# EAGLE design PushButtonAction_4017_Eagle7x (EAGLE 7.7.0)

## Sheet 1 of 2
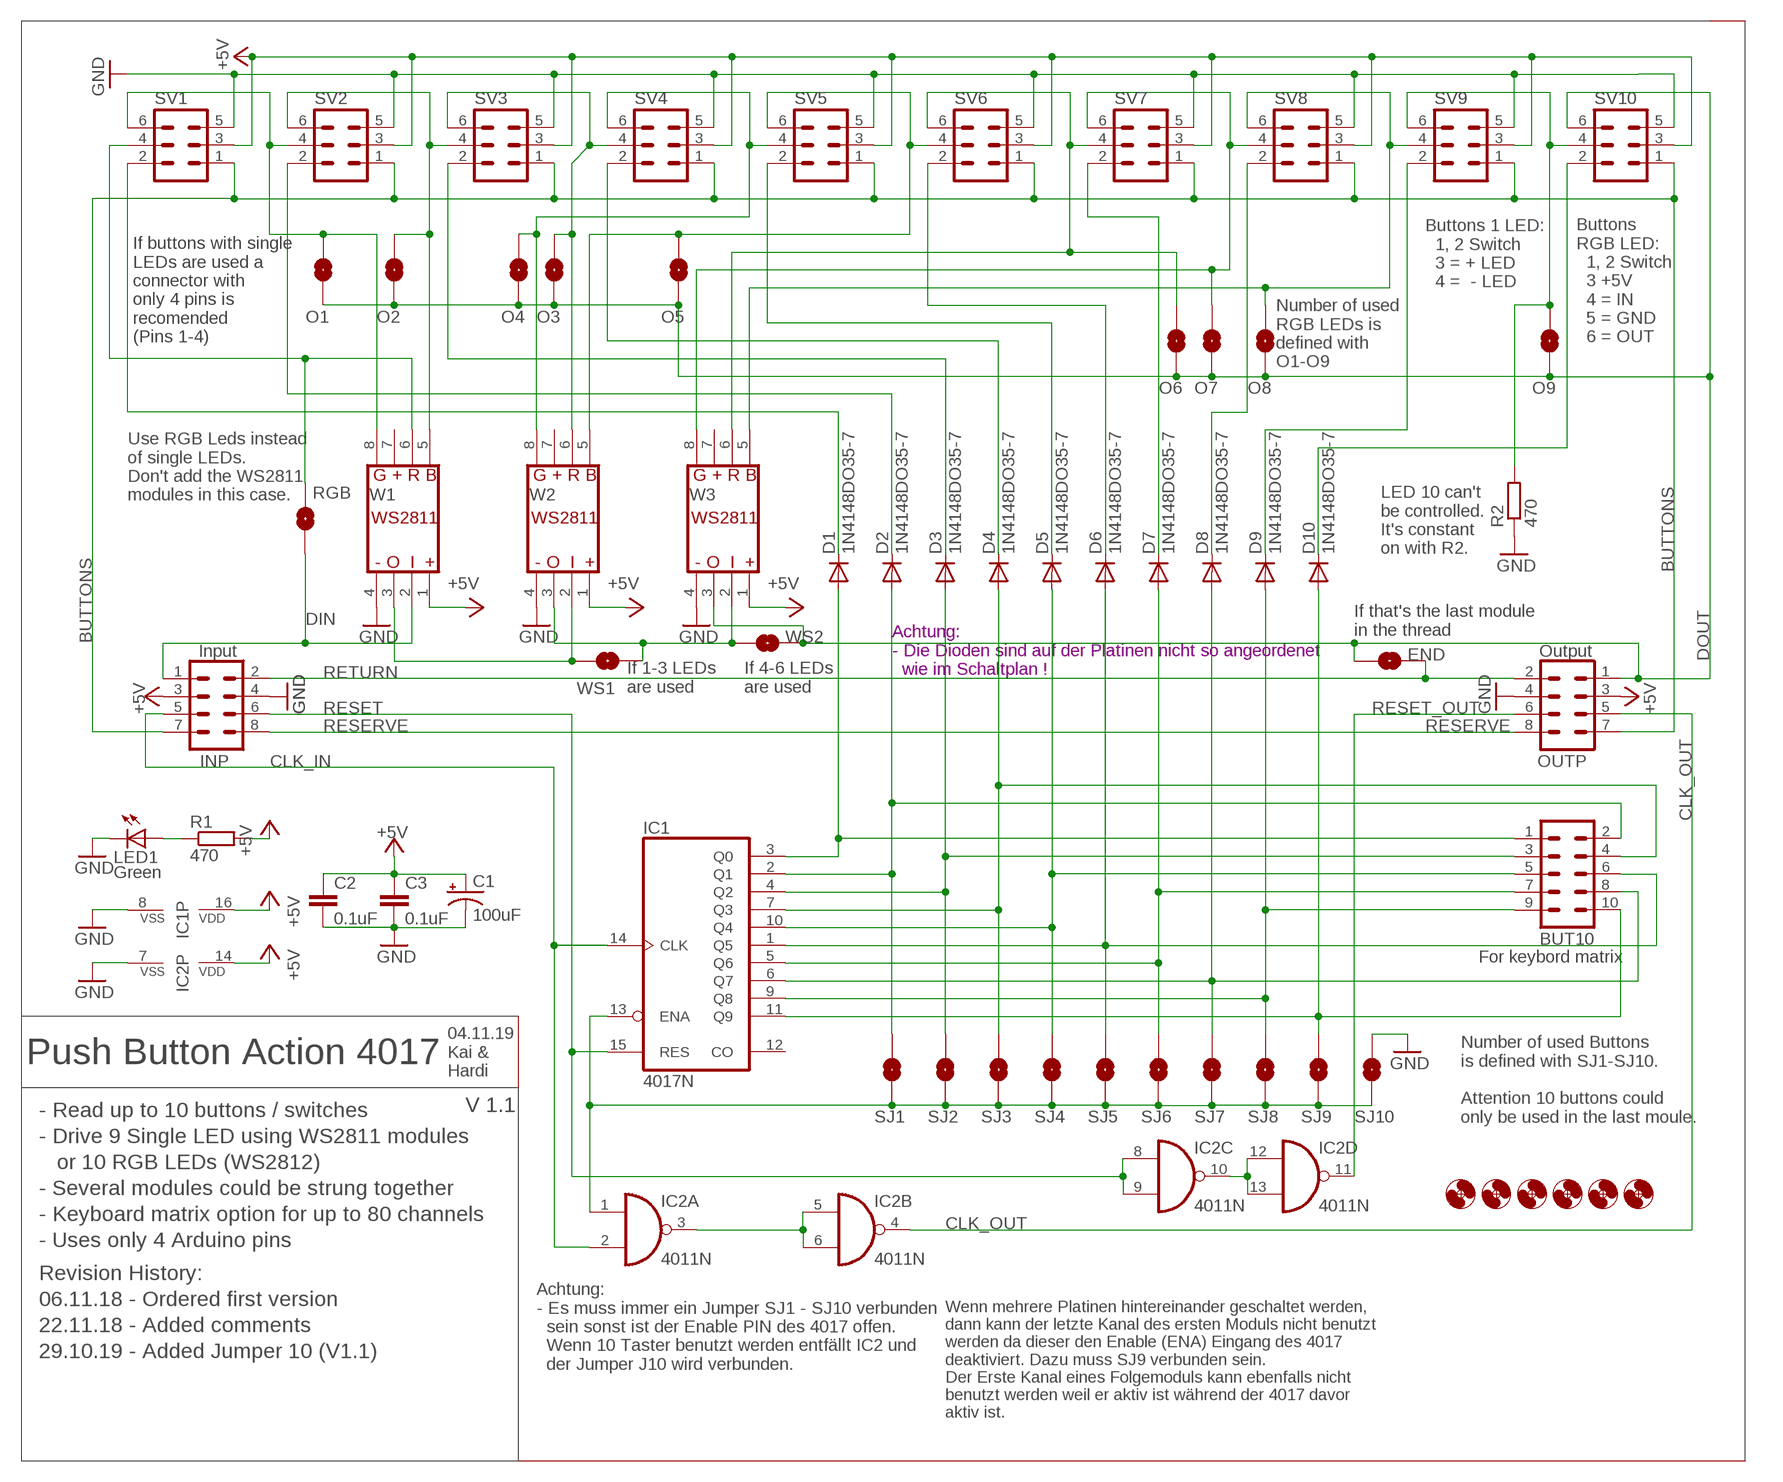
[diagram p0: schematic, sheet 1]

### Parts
BUT10  CON-HARTING-ML_ML10  [CON-HARTING-ML_ML10]
C1  100uF  100UF-25V-20%(PTH)  [CPOL-RADIAL-100UF-25V]
C2  0.1uF  0.1UF-50V-20%(PTH)KIT-EZ  [CAP-PTH-SMALL-KIT]
C3  0.1uF  0.1UF-50V-20%(PTH)KIT-EZ  [CAP-PTH-SMALL-KIT]
D1  1N4148DO35-7  [DO35-7]
D2  1N4148DO35-7  [DO35-7]
D3  1N4148DO35-7  [DO35-7]
D4  1N4148DO35-7  [DO35-7]
D5  1N4148DO35-7  [DO35-7]
D6  1N4148DO35-7  [DO35-7]
D7  1N4148DO35-7  [DO35-7]
D8  1N4148DO35-7  [DO35-7]
D9  1N4148DO35-7  [DO35-7]
D10  1N4148DO35-7  [DO35-7]
END  SOLDERJUMPERNO  [SJ_2S-NO]
H1  MOUNT-HOLE3.0  [3,0]
H2  MOUNT-HOLE3.0  [3,0]
H3  MOUNT-HOLE3.0  [3,0]
H4  MOUNT-HOLE3.0  [3,0]
H5  MOUNT-HOLE3.0  [3,0]
H6  MOUNT-HOLE3.0  [3,0]
IC1  4017N  [DIL16]
IC2  4011N  [DIL14]
INP  CON-HARTING-ML_ML08  [CON-HARTING-ML_ML08]
LED1  Green  LED3MM  [LED3MM]
O1  SOLDERJUMPERNO  [SJ_2S-NO]
O2  SOLDERJUMPERNO  [SJ_2S-NO]
O3  SOLDERJUMPERNO  [SJ_2S-NO]
O4  SOLDERJUMPERNO  [SJ_2S-NO]
O5  SOLDERJUMPERNO  [SJ_2S-NO]
O6  SOLDERJUMPERNO  [SJ_2S-NO]
O7  SOLDERJUMPERNO  [SJ_2S-NO]
O8  SOLDERJUMPERNO  [SJ_2S-NO]
O9  SOLDERJUMPERNO  [SJ_2S-NO]
OUTP  CON-HARTING-ML_ML08  [CON-HARTING-ML_ML08]
R1  470  R-EU_0207/2V  [0207/2V]
R2  470  R-EU_0204/5  [0204/5]
RGB  SOLDERJUMPERNO  [SJ_2S-NO]
SJ1  SOLDERJUMPERNO  [SJ_2S-NO]
SJ2  SOLDERJUMPERNO  [SJ_2S-NO]
SJ3  SOLDERJUMPERNO  [SJ_2S-NO]
SJ4  SOLDERJUMPERNO  [SJ_2S-NO]
SJ5  SOLDERJUMPERNO  [SJ_2S-NO]
SJ6  SOLDERJUMPERNO  [SJ_2S-NO]
SJ7  SOLDERJUMPERNO  [SJ_2S-NO]
SJ8  SOLDERJUMPERNO  [SJ_2S-NO]
SJ9  SOLDERJUMPERNO  [SJ_2S-NO]
SJ10  SOLDERJUMPERNO  [SJ_2S-NO]
SV1  CON-HARTING-ML_ML6  [CON-HARTING-ML_ML6]
SV2  CON-HARTING-ML_ML6  [CON-HARTING-ML_ML6]
SV3  CON-HARTING-ML_ML6  [CON-HARTING-ML_ML6]
SV4  CON-HARTING-ML_ML6  [CON-HARTING-ML_ML6]
SV5  CON-HARTING-ML_ML6  [CON-HARTING-ML_ML6]
SV6  CON-HARTING-ML_ML6  [CON-HARTING-ML_ML6]
SV7  CON-HARTING-ML_ML6  [CON-HARTING-ML_ML6]
SV8  CON-HARTING-ML_ML6  [CON-HARTING-ML_ML6]
SV9  CON-HARTING-ML_ML6  [CON-HARTING-ML_ML6]
SV10  CON-HARTING-ML_ML6  [CON-HARTING-ML_ML6]
W1  WS28115V  [WS2811_WS2811_5V]
W2  WS28115V  [WS2811_WS2811_5V]
W3  WS28115V  [WS2811_WS2811_5V]
WS1  SOLDERJUMPERNO  [SJ_2S-NO]
WS2  SOLDERJUMPERNO  [SJ_2S-NO]

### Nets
+5V: C1.1(+) C2.1 C3.1 IC1.16(VDD) IC2.14(P:VDD) INP.3 OUTP.3 R1.2 SV1.3 SV2.3 SV3.3 SV4.3 SV5.3 SV6.3 SV7.3 SV8.3 SV9.3 SV10.3 W1.1 W2.1 W3.1
BUTTONS: INP.7 OUTP.7 SV1.1 SV2.1 SV3.1 SV4.1 SV5.1 SV6.1 SV7.1 SV8.1 SV9.1 SV10.1
CLK_IN: IC1.14(CLK) IC2.2(A:I1) INP.5
CLK_OUT: IC2.4(B:O) OUTP.5
DIN: INP.1 RGB.1 W1.2
DOUT: END.2 O1.1 O2.1 O3.1 O4.1 O5.1 O6.1 O7.1 O8.1 O9.1 OUTP.1 SV10.6 W3.3 WS2.1
GND: C1.2(-) C2.2 C3.2 IC1.8(VSS) IC2.7(P:VSS) INP.4 LED1.K(C) OUTP.4 R2.1 SJ10.2 SV1.5 SV2.5 SV3.5 SV4.5 SV5.5 SV6.5 SV7.5 SV8.5 SV9.5 SV10.5 W1.4 W2.4 W3.4
N$1: IC2.3(A:O) IC2.5(B:I0) IC2.6(B:I1)
N$2: IC1.13(ENA) IC2.1(A:I0) SJ1.1 SJ2.1 SJ3.1 SJ4.1 SJ5.1 SJ6.1 SJ7.1 SJ8.1 SJ9.1 SJ10.1
N$3: IC2.10(C:O) IC2.12(D:I0) IC2.13(D:I1)
N$4: RGB.2 SV1.4 W1.6
N$5: BUT10.10 D10.A IC1.11(Q9) SJ9.2
N$6: D1.C SV1.2
N$7: W1.3 W2.2 WS1.1
N$8: O5.2 SV5.6 SV6.4 W2.5
N$9: D2.C SV2.2
N$10: D3.C SV3.2
N$11: BUT10.2 D2.A IC1.2(Q1) SJ1.2
N$12: BUT10.3 D3.A IC1.4(Q2) SJ2.2
N$13: BUT10.4 D4.A IC1.7(Q3) SJ3.2
N$14: BUT10.5 D5.A IC1.10(Q4) SJ4.2
N$15: BUT10.6 D6.A IC1.1(Q5) SJ5.2
N$16: BUT10.7 D7.A IC1.5(Q6) SJ6.2
N$17: BUT10.8 D8.A IC1.6(Q7) SJ7.2
N$18: BUT10.9 D9.A IC1.9(Q8) SJ8.2
N$19: D4.C SV4.2
N$20: D5.C SV5.2
N$21: LED1.A R1.1
N$22: W2.3 W3.2 WS1.2 WS2.2
N$23: D6.C SV6.2
N$25: D8.C SV8.2
N$26: D9.C SV9.2
N$27: D10.C SV10.2
N$35: BUT10.1 D1.A IC1.3(Q0)
N$45: O1.2 SV1.6 SV2.4 W1.8
N$46: O2.2 SV2.6 SV3.4 W1.5
N$49: O4.2 SV4.6 SV5.4 W2.8
N$51: O3.2 SV3.6 SV4.4 W2.6
N$54: O6.2 SV6.6 SV7.4 W3.6
N$56: O7.2 SV7.6 SV8.4 W3.8
N$57: O8.2 SV8.6 SV9.4 W3.5
N$58: O9.2 R2.2 SV9.6 SV10.4
O6: D7.C SV7.2
RESERVE: INP.8 OUTP.8
RESET: IC1.15(RES) IC2.8(C:I0) IC2.9(C:I1) INP.6
RESET_OUT: IC2.11(D:O) OUTP.6
RETURN: END.1 INP.2 OUTP.2
Unconnected: IC1.12(CO) W1.7 W2.7 W3.7

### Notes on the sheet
- Buttons 1 LED:
    1, 2 Switch
    3 = + LED
    4 =  - LED
- If buttons with single 
  LEDs are used a 
  connector with
  only 4 pins is 
  recomended
  (Pins 1-4)
- Buttons
  RGB LED:
    1, 2 Switch
    3 +5V
    4 = IN
    5 = GND
    6 = OUT
- Number of used
  RGB LEDs is 
  defined with 
  O1-O9
- Use RGB Leds instead
  of single LEDs.
  Don't add the WS2811
  modules in this case.
- LED 10 can't
  be controlled.
  It's constant
  on with R2.
- Achtung:
  - Die Dioden sind auf der Platinen nicht so angeordenet
    wie im Schaltplan !
- If that's the last module 
  in the thread
- Input | Output
- If 1-3 LEDs
  are used
- If 4-6 LEDs
  are used
- For keybord matrix
- Push Button Action 4017
- 04.11.19
  Kai & 
  Hardi
- V 1.1
- Number of used Buttons
  is defined with SJ1-SJ10.
  
  Attention 10 buttons could
  only be used in the last moule.
- - Read up to 10 buttons / switches
  - Drive 9 Single LED using WS2811 modules
     or 10 RGB LEDs (WS2812)
  - Several modules could be strung together
  - Keyboard matrix option for up to 80 channels
  - Uses only 4 Arduino pins
- Revision History:
  06.11.18 - Ordered first version
  22.11.18 - Added comments
  29.10.19 - Added Jumper 10 (V1.1)
- Achtung:
  - Es muss immer ein Jumper SJ1 - SJ10 verbunden
    sein sonst ist der Enable PIN des 4017 offen.
    Wenn 10 Taster benutzt werden entfällt IC2 und 
    der Jumper J10 wird verbunden.
- Wenn mehrere Platinen hintereinander geschaltet werden,
  dann kann der letzte Kanal des ersten Moduls nicht benutzt
  werden da dieser den Enable (ENA) Eingang des 4017
  deaktiviert. Dazu muss SJ9 verbunden sein.
  Der Erste Kanal eines Folgemoduls kann ebenfalls nicht
  benutzt werden weil er aktiv ist während der 4017 davor
  aktiv ist.

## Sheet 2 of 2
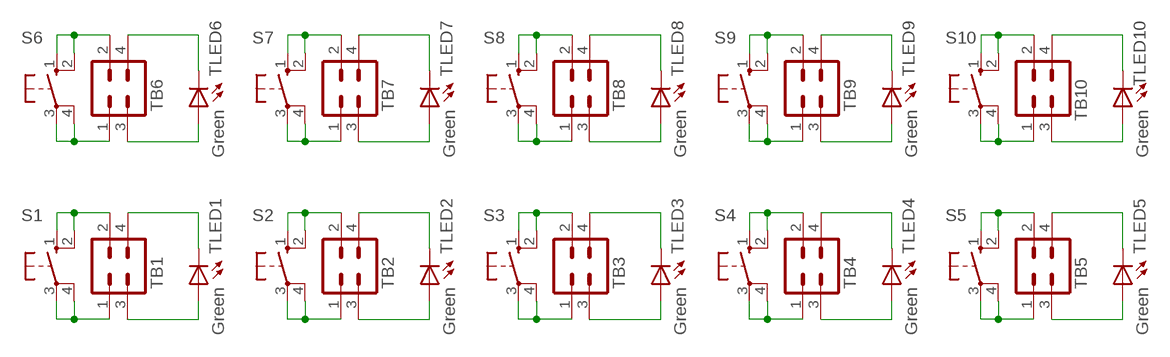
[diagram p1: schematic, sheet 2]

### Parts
S1  10-XX  [B3F-10XX]
S2  10-XX  [B3F-10XX]
S3  10-XX  [B3F-10XX]
S4  10-XX  [B3F-10XX]
S5  10-XX  [B3F-10XX]
S6  10-XX  [B3F-10XX]
S7  10-XX  [B3F-10XX]
S8  10-XX  [B3F-10XX]
S9  10-XX  [B3F-10XX]
S10  10-XX  [B3F-10XX]
TB1  CON-HARTING-ML_ML4ML4_FEMALE  [ML_ML4_FEMALE]
TB2  CON-HARTING-ML_ML4ML4_FEMALE  [ML_ML4_FEMALE]
TB3  CON-HARTING-ML_ML4ML4_FEMALE  [ML_ML4_FEMALE]
TB4  CON-HARTING-ML_ML4ML4_FEMALE  [ML_ML4_FEMALE]
TB5  CON-HARTING-ML_ML4ML4_FEMALE  [ML_ML4_FEMALE]
TB6  CON-HARTING-ML_ML4ML4_FEMALE  [ML_ML4_FEMALE]
TB7  CON-HARTING-ML_ML4ML4_FEMALE  [ML_ML4_FEMALE]
TB8  CON-HARTING-ML_ML4ML4_FEMALE  [ML_ML4_FEMALE]
TB9  CON-HARTING-ML_ML4ML4_FEMALE  [ML_ML4_FEMALE]
TB10  CON-HARTING-ML_ML4ML4_FEMALE  [ML_ML4_FEMALE]
TLED1  Green  LED_LED3MM  [LED_LED3MM]
TLED2  Green  LED_LED3MM  [LED_LED3MM]
TLED3  Green  LED_LED3MM  [LED_LED3MM]
TLED4  Green  LED_LED3MM  [LED_LED3MM]
TLED5  Green  LED_LED3MM  [LED_LED3MM]
TLED6  Green  LED_LED3MM  [LED_LED3MM]
TLED7  Green  LED_LED3MM  [LED_LED3MM]
TLED8  Green  LED_LED3MM  [LED_LED3MM]
TLED9  Green  LED_LED3MM  [LED_LED3MM]
TLED10  Green  LED_LED3MM  [LED_LED3MM]

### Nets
N$24: S1.1(S) S1.2(S1) TB1.2
N$28: S1.3(P) S1.4(P1) TB1.1
N$29: TB1.3 TLED1.A
N$30: TB1.4 TLED1.K(C)
N$31: S2.1(S) S2.2(S1) TB2.2
N$32: S2.3(P) S2.4(P1) TB2.1
N$33: TB2.3 TLED2.A
N$34: TB2.4 TLED2.K(C)
N$36: S3.1(S) S3.2(S1) TB3.2
N$37: S3.3(P) S3.4(P1) TB3.1
N$38: TB3.3 TLED3.A
N$39: TB3.4 TLED3.K(C)
N$40: S4.1(S) S4.2(S1) TB4.2
N$41: S4.3(P) S4.4(P1) TB4.1
N$42: TB4.3 TLED4.A
N$43: TB4.4 TLED4.K(C)
N$44: S5.1(S) S5.2(S1) TB5.2
N$47: S5.3(P) S5.4(P1) TB5.1
N$48: TB5.3 TLED5.A
N$50: TB5.4 TLED5.K(C)
N$52: S6.1(S) S6.2(S1) TB6.2
N$53: S6.3(P) S6.4(P1) TB6.1
N$55: TB6.3 TLED6.A
N$59: TB6.4 TLED6.K(C)
N$60: S7.1(S) S7.2(S1) TB7.2
N$61: S7.3(P) S7.4(P1) TB7.1
N$62: TB7.3 TLED7.A
N$63: TB7.4 TLED7.K(C)
N$64: S8.1(S) S8.2(S1) TB8.2
N$65: S8.3(P) S8.4(P1) TB8.1
N$66: TB8.3 TLED8.A
N$67: TB8.4 TLED8.K(C)
N$68: S9.1(S) S9.2(S1) TB9.2
N$69: S9.3(P) S9.4(P1) TB9.1
N$70: TB9.3 TLED9.A
N$71: TB9.4 TLED9.K(C)
N$72: S10.1(S) S10.2(S1) TB10.2
N$73: S10.3(P) S10.4(P1) TB10.1
N$74: TB10.3 TLED10.A
N$75: TB10.4 TLED10.K(C)

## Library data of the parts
BUT10 = PushButtonAction_4017_2:CON-HARTING-ML_ML10: HARTING; OC_FARNELL: unknown; OC_NEWARK: unknown
C1 = SparkFun-Capacitors:100UF-25V-20%(PTH): CAP-08439; PROD_ID: CAP-08439
C2 C3 = SparkFun-Capacitors:0.1UF-50V-20%(PTH): CAP-08370; PROD_ID: CAP-08370
D1-D10 = diode:1N4148: DIODE
END O1-O9 RGB SJ1-SJ10 WS1 WS2 = SparkFun-Retired:SOLDERJUMPER: Solder Jumper
H1-H6 = holes:MOUNT-HOLE: MOUNTING HOLE with drill center marker
IC1 = 40xx:4017: COUNTER/DIVIDER
IC2 = 40xx:4011: Quad 2-input NAND; SPICEPREFIX: J
INP OUTP = PushButtonAction_4017_2:CON-HARTING-ML_ML08: Modified by Hardi; OC_FARNELL: unknown; OC_NEWARK: unknown
LED1 = led:LED: LED
R1 R2 = rcl:R-EU_: RESISTOR, European symbol; SPICEPREFIX: R
S1-S10 = switch-omron:10-XX: OMRON SWITCH; MPN: B3F-1000; OC_FARNELL: 176432; OC_NEWARK: 36M3542
SV1-SV10 = PushButtonAction_4017_4:CON-HARTING-ML_ML6: HARTING; OC_FARNELL: unknown; OC_NEWARK: unknown
TB1-TB10 = RGB-LED-Verteiler:CON-HARTING-ML_ML4
TLED1-TLED10 = Sound_MP3-TF-16P_and_WS2811:LED_LED: LED
W1-W3 = PushButtonAction_4017_2:WS2811: Modified by Hardi

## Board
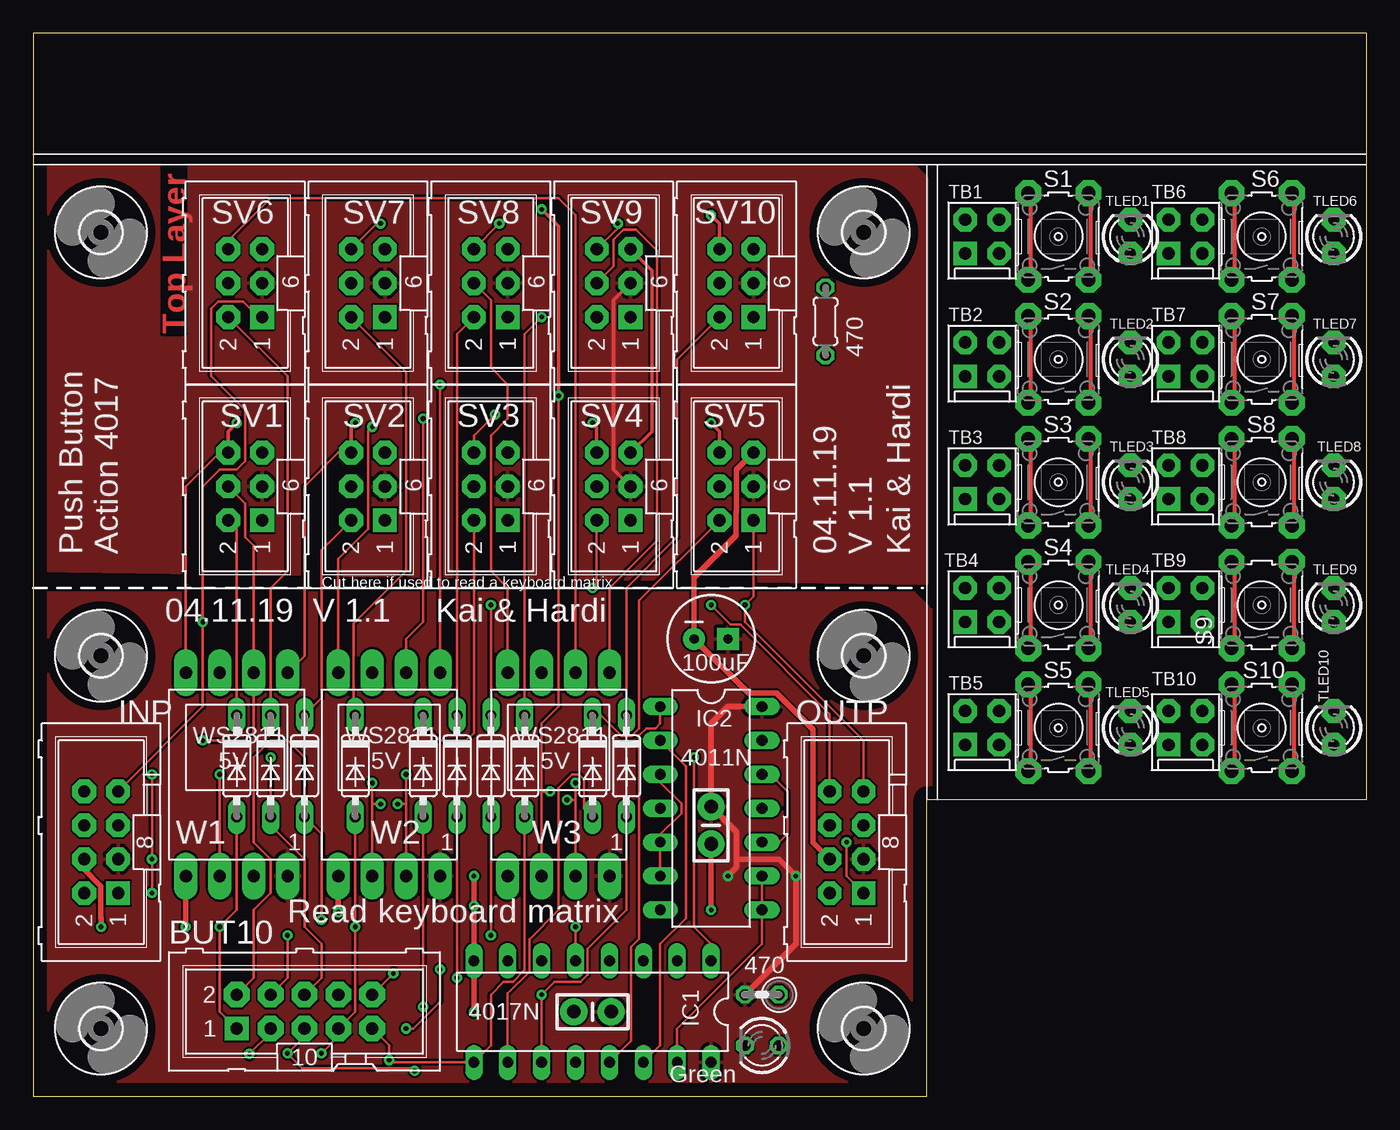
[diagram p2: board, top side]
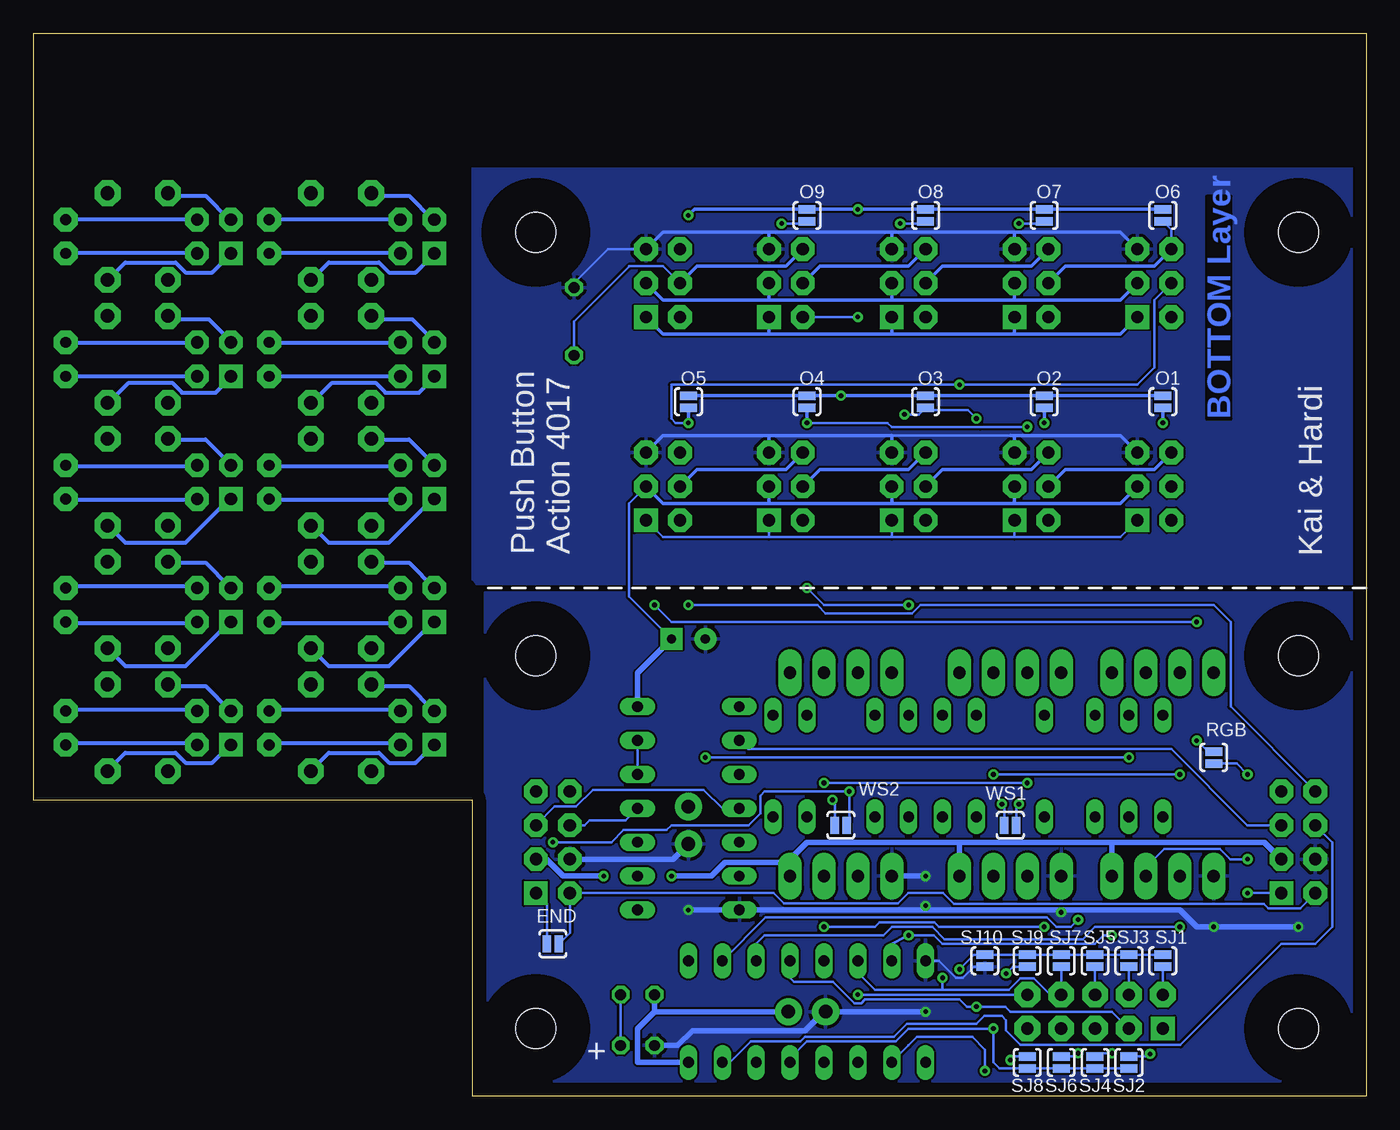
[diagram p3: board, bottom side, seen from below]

Size 99.9 x 79.68 mm. Coordinates in mm from the lower left corner, seen from the top.
Outline: 0,0 66.98,0 66.98,22.23 99.9,22.23 99.9,79.68 0,79.68 0,0
Copper layers (1*16): Top 0.035mm / dielectric 1.5mm / Bottom 0.035mm
Design rules "default *": minimum track width 6mil, minimum drill 0.35mm, track to track 6mil, track to pad 6mil, pad to pad 6mil, via to via 6mil, smd to smd 6mil, copper to edge 40mil, drill to drill 6mil, minimum pad ring 10mil, minimum via ring 8mil, stop-mask expansion 4mil, vias tented up to drill 0mil, thermal gap 10mil

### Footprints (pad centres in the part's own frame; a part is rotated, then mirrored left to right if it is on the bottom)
CON-HARTING-ML_ML10 = drill 0.914 pad 1.778 square: 1 -5.08,-1.27 | drill 0.914 pad 1.93 octagon: 2 -5.08,1.27; 3 -2.54,-1.27; 4 -2.54,1.27; 5 0,-1.27; 6 0,1.27; 7 2.54,-1.27; 8 2.54,1.27; 9 5.08,-1.27; 10 5.08,1.27
CPOL-RADIAL-100UF-25V = drill 0.7 pad 1.651 square: 1 1.27,0 | drill 0.7 pad 1.651: 2 -1.27,0
CAP-PTH-SMALL-KIT = drill 1.016 pad 2.032: 1 -1.397,0; 2 1.397,0
DO35-7 = drill 0.813 long: A 3.81,0; C -3.81,0
SJ_2S-NO = smd 0.635 x 1.27: 1 -0.45,0; 2 0.45,0
3,0 = hole 3: 0,0
DIL16 = drill 0.813 long: 1 -8.89,-3.81; 2 -6.35,-3.81; 3 -3.81,-3.81; 4 -1.27,-3.81; 5 1.27,-3.81; 6 3.81,-3.81; 7 6.35,-3.81; 8 8.89,-3.81; 9 8.89,3.81; 10 6.35,3.81; 11 3.81,3.81; 12 1.27,3.81; 13 -1.27,3.81; 14 -3.81,3.81; 15 -6.35,3.81; 16 -8.89,3.81
DIL14 = drill 0.813 long: 1 -7.62,-3.81; 2 -5.08,-3.81; 3 -2.54,-3.81; 4 0,-3.81; 5 2.54,-3.81; 6 5.08,-3.81; 7 7.62,-3.81; 8 7.62,3.81; 9 5.08,3.81; 10 2.54,3.81; 11 0,3.81; 12 -2.54,3.81; 13 -5.08,3.81; 14 -7.62,3.81
CON-HARTING-ML_ML08 = drill 0.914 pad 1.778 square: 1 -5.08,-1.27 | drill 0.914 pad 1.778 octagon: 2 -5.08,1.27; 3 -2.54,-1.27; 4 -2.54,1.27; 5 0,-1.27; 6 0,1.27; 7 2.54,-1.27; 8 2.54,1.27
LED3MM = drill 0.813 octagon: A -1.27,0; K 1.27,0
0207/2V = drill 0.813 octagon: 1 -1.27,0; 2 1.27,0
0204/5 = drill 0.813 octagon: 1 -2.54,0; 2 2.54,0
B3F-10XX = drill 1.016 pad 1.93 octagon: 1 -3.251,2.261; 2 3.251,2.261; 3 -3.251,-2.261; 4 3.251,-2.261
CON-HARTING-ML_ML6 = drill 0.914 pad 1.778 square: 1 -2.54,-1.27 | drill 0.914 pad 1.778 octagon: 2 -2.54,1.27; 3 0,-1.27; 4 0,1.27; 5 2.54,-1.27; 6 2.54,1.27
ML_ML4_FEMALE = drill 0.914 pad 1.778 square: 1 -2.54,-1.27 | drill 0.914 pad 1.778 octagon: 2 -2.54,1.27; 3 0,-1.27; 4 0,1.27
LED_LED3MM = drill 0.813 pad 1.778 octagon: A -1.27,0; K 1.27,0
WS2811_WS2811_5V = drill 0.914 pad 1.778 long: 1 2.54,-5.08; 2 0,-5.08; 3 -2.54,-5.08; 4 -5.08,-5.08; 5 2.54,10.16; 6 0,10.16; 7 -2.54,10.16; 8 -5.08,10.16

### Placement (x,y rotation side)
BUT10  20.32,6.35 0 top
C1  50.8,34.29 0 top
C2  50.8,20.32 270 top
C3  41.91,6.35 180 top
D1  15.24,24.77 270 top
D2  20.32,24.77 270 top
D3  29.21,24.77 270 top
D4  34.29,24.77 270 top
D5  41.91,24.77 270 top
D6  17.78,24.77 270 top
D7  24.13,24.77 270 top
D8  31.75,24.77 270 top
D9  36.83,24.77 270 top
D10  44.45,24.77 270 top
END  60.96,11.43 180 bottom
H1  62.23,5.08 90 top
H2  5.08,5.08 90 top
H3  5.08,64.77 90 top
H4  62.23,64.77 90 top
H5  5.08,33.02 90 top
H6  62.23,33.02 90 top
IC1  41.91,6.35 180 top
IC2  50.8,21.59 270 top
INP  5.08,20.32 90 top
LED1  54.61,3.81 180 top
O1  15.24,52.07 270 bottom
O2  24.13,52.07 270 bottom
O3  33.02,52.07 270 bottom
O4  41.91,52.07 270 bottom
O5  50.8,52.07 270 bottom
O6  15.24,66.04 270 bottom
O7  24.13,66.04 270 bottom
O8  33.02,66.04 270 bottom
O9  41.91,66.04 270 bottom
OUTP  60.96,20.32 90 top
R1  54.61,7.62 180 top
R2  59.37,58.09 270 top
RGB  11.43,25.4 90 bottom
S1  76.83,64.45 90 top
S2  76.83,55.24 90 top
S3  76.83,46.04 90 top
S4  76.83,36.83 90 top
S5  76.83,27.62 90 top
S6  92.08,64.45 90 top
S7  92.08,55.24 90 top
S8  92.08,46.04 90 top
S9  92.08,36.83 90 top
S10  92.08,27.62 90 top
SJ1  15.24,10.16 270 bottom
SJ2  17.78,2.54 90 bottom
SJ3  17.78,10.16 270 bottom
SJ4  20.32,2.54 90 bottom
SJ5  20.32,10.16 270 bottom
SJ6  22.86,2.54 90 bottom
SJ7  22.86,10.16 270 bottom
SJ8  25.4,2.54 90 bottom
SJ9  25.4,10.16 270 bottom
SJ10  28.57,10.16 270 bottom
SV1  15.88,45.72 90 top
SV2  25.08,45.72 90 top
SV3  34.29,45.72 90 top
SV4  43.5,45.72 90 top
SV5  52.7,45.72 90 top
SV6  15.88,60.96 90 top
SV7  25.08,60.96 90 top
SV8  34.29,60.96 90 top
SV9  43.5,60.96 90 top
SV10  52.7,60.96 90 top
TB1  72.39,64.45 0 top
TB2  72.39,55.24 0 top
TB3  72.39,46.04 0 top
TB4  72.39,36.83 0 top
TB5  72.39,27.62 0 top
TB6  87.63,64.45 0 top
TB7  87.63,55.24 0 top
TB8  87.63,46.04 0 top
TB9  87.63,36.83 0 top
TB10  87.63,27.62 0 top
TLED1  82.23,64.45 90 top
TLED2  82.23,55.24 90 top
TLED3  82.23,46.04 90 top
TLED4  82.23,36.83 90 top
TLED5  82.23,27.62 90 top
TLED6  97.47,64.45 90 top
TLED7  97.47,55.24 90 top
TLED8  97.47,46.04 90 top
TLED9  97.47,36.83 90 top
TLED10  97.47,27.62 90 top
W1  16.51,21.59 0 top
W2  27.94,21.59 0 top
W3  40.64,21.59 0 top
WS1  26.67,20.32 0 bottom
WS2  39.37,20.32 180 bottom

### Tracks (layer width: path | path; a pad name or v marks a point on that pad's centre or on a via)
+5V  (via drill 0.35)
  Top 0.254: SV9.3 43.5,59.69 43.5,46.99 SV4.3
  Top 0.406: IC2.14 52.07,29.21 50.8,27.94 C2.1 52.7,19.81 52.7,17.78 | R1.2 57.15,11.43 v57.15,16.51 55.88,17.78 52.7,17.78 | 52.7,17.78 52.7,17.14 v52.07,16.51
  Bottom 0.203: SV5.3 55.24,44.45 55.24,37.47 C1.1
  Bottom 0.254: SV6.3 18.41,59.69 26.35,59.69 | 26.35,59.69 35.56,59.69 | 35.56,59.69 44.77,59.69 | 44.77,59.69 52.7,59.69 SV10.3 | SV7.3 26.35,59.69 | SV8.3 35.56,59.69 | SV9.3 44.77,59.69 | SV1.3 18.41,44.45 26.35,44.45 | 26.35,44.45 35.56,44.45 | 35.56,44.45 44.77,44.45 | 44.77,44.45 52.7,44.45 SV5.3 | SV2.3 26.35,44.45 | SV3.3 35.56,44.45 | SV4.3 44.77,44.45
  Bottom 0.406: 19.05,19.05 7.62,19.05 INP.3 | 19.05,19.05 30.48,19.05 | 30.48,19.05 41.91,19.05 43.18,17.78 | OUTP.3 61.45,17.78 60.21,16.54 57.17,16.54 v57.15,16.51 | v52.07,16.51 49.09,16.51 48.07,17.53 43.43,17.53 43.18,17.78 | 53.34,6.35 R1.2 | C3.1 53.34,6.35 | 53.34,6.35 54.61,5.08 54.61,2.54 IC1.16 | C1.1 54.61,31.75 IC2.14 | W1.1 19.05,19.05 | W3.1 43.18,17.78 | W2.1 30.48,19.05
  pour Top: 0,0 67.31,0 67.31,36.51 66.04,37.78 0.95,37.78 0,1.27
  pour Top: 66.99,38.42 66.99,68.9 66.04,69.85 1.27,69.85 0,68.58 0,39.37
BUTTONS  (via drill 0.35)
  Top 0.203: INP.7 12.7,29.21 v12.7,35.56 12.7,45.72 13.97,46.99 15.24,46.99 15.88,47.62 15.88,51.44 13.34,53.98 13.34,59.05 13.84,59.56 15.71,59.56 16.86,58.42 SV6.1 | SV5.1 53.98,37.47 v53.34,36.83 53.34,35.56 62.23,26.67 OUTP.7
  Bottom 0.203: SV1.1 18.41,41.91 26.35,41.91 | 26.35,41.91 35.56,41.91 | 35.56,41.91 44.77,41.91 | 44.77,41.91 52.7,41.91 SV5.1 | SV2.1 26.35,41.91 | SV3.1 35.56,41.91 | SV4.1 44.77,41.91 | v12.7,35.56 52.07,35.56 v53.34,36.83
  Bottom 0.254: SV6.1 18.41,57.15 26.35,57.15 | 26.35,57.15 35.56,57.15 | 35.56,57.15 44.77,57.15 | 44.77,57.15 52.7,57.15 SV10.1 | SV7.1 26.35,57.15 | SV8.1 35.56,57.15 | SV9.1 44.77,57.15
CLK_IN
  Top 0.203: IC2.2 48.9,24.77 48.92,24.74 48.92,13.36 46.99,11.43 46.99,3.81 IC1.14
  Bottom 0.203: INP.5 8.89,20.32 14.6,26.03 46.35,26.03 IC2.2
CLK_OUT
  Bottom 0.203: IC2.4 48.26,21.59 49.66,22.99 57.95,22.99 59.22,21.72 60.83,21.72 OUTP.5
DIN  (via drill 0.35)
  Top 0.203: v8.89,15.24 v8.89,17.78 v8.89,24.13
  Bottom 0.203: INP.1 7.62,15.24 v8.89,15.24 | v8.89,17.78 10.2,17.78 10.96,18.54 15.11,18.54 16.51,17.14 W1.2 | v8.89,24.13 9.71,24.95 RGB.1
DOUT  (via drill 0.35)
  Top 0.203: OUTP.1 60.96,16.51 v60.96,19.05 | 38.1,22.86 38.1,27.94 39.37,29.21 v39.37,52.52 | 38.1,22.86 v38.74,22.86 | W3.3 38.1,22.86
  Top 0.254: SV10.6 51.44,65.41 v50.8,66.04 | v39.37,52.52 39.37,65.22 v38.1,66.49
  Bottom 0.203: OUTP.1 61.41,14.42 END.2 | WS2.1 38.74,20.5 v38.74,22.86 45.09,22.86 45.41,22.53 45.41,21.21 46.31,20.32 52.07,20.32 52.43,19.96 55.65,19.96 56.56,19.05 v60.96,19.05
  Bottom 0.254: O6.1 O7.1 O8.1 v38.1,66.49 O9.1 50.35,66.49 v50.8,66.04 | O1.1 O2.1 | O1.1 O3.1 | v39.37,52.52 35.56,52.52 O1.1 | v39.37,52.52 O4.1 | v39.37,52.52 O5.1
GND  (via drill 0.35)
  Top 0.254: SV9.5 46.35,61.91 46.35,49.85 SV4.5
  Top 0.406: v33.02,6.35 IC1.8 v33.02,14.29 v33.02,16.51 | INP.4 3.81,17 5.05,15.76 5.05,13.36 5.08,13.34 v5.08,12.7 | 22.86,13.65 v22.86,13.79 W2.4 | C2.2 v50.8,13.97 | SV5.5 52.7,46.99 52.7,43.81 52.68,43.79 52.68,42.03 49.53,38.88 C1.2 53.59,30.23 55.69,30.23 58.42,27.5 58.42,19.05 OUTP.4 | W1.4 v11.43,12.7
  Bottom 0.203: 35.56,49.53 26.67,49.53 | SV10.5 56.83,63.5 59.37,60.96 R2.1 | SJ10.2 29.4,9.71 30.22,8.89 30.74,8.89 32.01,10.16 IC1.8
  Bottom 0.254: SV6.5 18.41,64.77 26.35,64.77 | SV10.5 52.7,64.77 44.77,64.77 | 26.35,64.77 35.56,64.77 | 35.56,64.77 44.77,64.77 | 26.35,64.77 SV7.5 | 35.56,64.77 SV8.5 | 44.77,64.77 SV9.5 | SV1.5 18.41,49.53 26.35,49.53 | 26.35,49.53 26.67,49.53 | 44.77,49.53 35.56,49.53 SV3.5 | 44.77,49.53 52.7,49.53 SV5.5 | SV2.5 26.35,49.53 | SV4.5 44.77,49.53
  Bottom 0.406: 33.02,13.97 IC2.7 v50.8,13.97 | v33.02,14.29 33.02,13.97 | 33.02,13.97 22.86,13.97 | 22.86,13.97 13.97,13.97 12.7,12.7 v11.43,12.7 v5.08,12.7 | v22.86,13.79 22.86,13.97 | v33.02,6.35 C3.2 40.64,6.35 42.06,4.93 50.51,4.93 51.63,3.81 LED1.K | OUTP.4 51.94,17.78 C2.2 | W3.4 v33.02,16.51
  pour Bottom: 0,0 66.04,0 66.04,37.78 0,37.78
  pour Bottom: 0,38.42 66.67,38.42 66.99,38.73 66.99,69.53 0.95,69.53
N$1
  Top 0.203: IC2.6 IC2.5 46.99,19.64 48.56,21.21 48.56,21.97 46.99,23.54 IC2.3
N$2  (via drill 0.35)
  Top 0.203: IC1.13 44.81,4.17 44.81,11.2 45.41,11.81 45.41,27.05 45.95,27.58 46.63,27.58 46.99,27.94 IC2.1 | v30.48,9.53 30.48,7.09 28.47,5.08 v27.94,5.08
  Bottom 0.203: SJ1.1 SJ3.1 SJ5.1 SJ7.1 SJ9.1 SJ10.1 29.39,10.61 v30.48,9.53 | SJ2.1 SJ4.1 SJ6.1 SJ8.1 27.49,2.09 27.94,2.54 v27.94,5.08 34.29,5.08 35.26,4.12 41.91,4.12 43.18,2.85 IC1.13
N$3
  Top 0.203: IC2.10 55.88,19.05 56.52,19.68 56.52,22.86 55.24,24.13 IC2.12
  Bottom 0.203: IC2.12 IC2.13
N$4  (via drill 0.35)
  Top 0.203: v12.7,26.67 15.88,26.67 16.51,27.3 W1.6 16.51,41.27 15.88,41.91 15.88,44.45 SV1.4
  Bottom 0.203: RGB.2 11.88,25.85 v12.7,26.67
N$5  (via drill 0.35)
  Top 0.203: IC1.11 v38.1,7.62 39.06,8.59 41.02,8.59 41.55,9.12 41.55,11.07 44.45,13.97 D10.A | BUT10.10 v26.99,9.21
  Bottom 0.203: BUT10.10 v38.1,7.62 | v26.99,9.21 26.48,9.71 SJ9.2
N$6
  Top 0.203: D1.C 15.24,42.55 SV1.2
N$7  (via drill 0.35)
  Top 0.203: 27.94,21.91 v27.94,24.13 | v27.3,21.91 27.94,21.91 | W1.3 v13.97,24.13 | W2.2 27.94,21.91
  Bottom 0.203: v13.97,24.13 v27.94,24.13 | WS1.1 27.12,21.72 v27.3,21.91
N$8  (via drill 0.35)
  Top 0.203: W2.5 v30.48,53.34
  Top 0.254: SV5.6 51.44,49.85 v50.8,50.48
  Bottom 0.203: v50.8,50.48 51.75,50.48 52.07,50.8 52.07,53.34 v30.48,53.34 17.14,53.34 15.88,54.61 15.88,59.69 SV6.4
  Bottom 0.254: v50.8,50.48 O5.2
N$9
  Top 0.203: D2.C 21.59,29.84 21.59,40.96 SV2.2
N$10
  Top 0.203: SV3.2 33.02,27.26 32.43,26.67 30.48,26.67 29.21,27.94 D3.C
N$11  (via drill 0.35)
  Top 0.203: BUT10.2 16.51,8.89 16.51,13.97 17.78,15.24 17.78,17.78 16.51,19.05 16.51,25.4 17.78,26.67 19.05,26.67 20.32,25.4 D2.A 21.59,19.68 v21.59,13.24
  Bottom 0.203: BUT10.2 SJ1.2 | IC1.2 45.01,13.41 23.95,13.41 23.24,12.7 22.13,12.7 v21.59,13.24
N$12  (via drill 0.35)
  Top 0.203: D3.A v29.21,6.72 | v16.19,3.17 17.78,4.76 BUT10.3
  Bottom 0.203: IC1.4 43.18,8.89 42.88,8.59 39.96,8.59 38.36,6.99 37.84,6.99 37.56,7.26 30.48,7.26 29.93,6.72 v29.21,6.72 27.04,6.72 26.67,6.35 19.05,6.35 BUT10.3 | SJ2.2 16.38,2.99 v16.19,3.17
N$13  (via drill 0.35)
  Top 0.203: BUT10.4 19.05,8.89 v19.05,12.06 | v34.29,12.06 D4.A
  Bottom 0.203: BUT10.4 SJ3.2 | v34.29,12.06 34.54,11.94 | 34.54,11.94 35.56,11.43 IC1.7 | v19.05,12.06 19.68,12.06 20.32,11.43 31.75,11.43 32.38,12.06 34.42,12.06 34.54,11.94
N$14  (via drill 0.35)
  Top 0.203: IC1.10 35.56,7.7 37.19,9.33 37.19,11.79 39.37,13.97 39.37,23.12 40.38,24.13 40.9,24.13 41.27,23.76 41.27,21.59 D5.A | BUT10.5 20.32,4.5 v19.05,3.23 19.05,3.17 20.14,2.09 26.67,2.09 28.39,2.09 v28.57,1.91
  Bottom 0.203: IC1.10 34.29,3.81 33.66,4.45 29.53,4.45 28.57,3.49 v28.57,1.91 | v19.05,3.23 20.08,3.23 SJ4.2
N$15  (via drill 0.35)
  Top 0.203: BUT10.6 21.59,8.89 21.59,11.43 20.32,12.7 20.32,17.78 17.78,20.32 D6.A v17.78,25.4 | IC1.1 50.8,11.43 49.53,12.7 v49.53,25.4
  Bottom 0.203: BUT10.6 SJ5.2 | v49.53,25.4 v17.78,25.4
N$16  (via drill 0.35)
  Top 0.203: D7.A v24.13,12.7 24.13,6.35 BUT10.7 22.86,4.5 v21.59,3.23 | v40.64,12.7 IC1.5
  Bottom 0.203: v24.13,12.7 32.01,12.7 32.37,13.06 36.47,13.06 36.83,12.7 v40.64,12.7 | SJ6.2 21.77,2.99 21.59,3.17 v21.59,3.23
N$17  (via drill 0.35)
  Top 0.203: v31.75,8.89 D8.A
  Bottom 0.203: SJ7.2 BUT10.8 23.68,7.62 24.89,8.84 25.91,8.84 26.77,7.98 31.75,7.98 | 31.75,7.98 36.83,7.98 38.1,9.25 IC1.6 | 31.75,7.98 v31.75,8.89
N$18  (via drill 0.35)
  Top 0.203: D9.A 36.83,9.48 35.94,8.59 35.26,8.59 34.29,7.62 34.29,3.81 IC1.9 26.67,2.54 v26.67,2.72 26.67,3.81 BUT10.9
  Bottom 0.203: v26.67,2.72 26.4,2.99 SJ8.2
N$19  (via drill 0.35)
  Top 0.203: D4.C v34.29,36.83 | SV4.2 42.23,38.42 v41.91,38.1
  Bottom 0.203: v34.29,36.83 40.64,36.83 v41.91,38.1
N$20
  Top 0.203: SV5.2 45.41,37.16 45.41,27.59 44.83,27 44.07,27 42.5,28.57 D5.C
N$21
  Bottom 0.203: LED1.A R1.1
N$22  (via drill 0.35)
  Top 0.203: v40.64,23.5 40.64,22.23 | 25.4,21.91 v25.4,23.5 | v40.01,22.23 40.64,22.23 | v26.04,21.91 25.4,21.91 | W2.3 25.4,21.91 | W3.2 40.64,22.23
  Bottom 0.203: v25.4,23.5 v40.64,23.5 | WS2.2 39.82,22.04 v40.01,22.23 | WS1.2 26.22,21.72 v26.04,21.91
N$23
  Top 0.203: D6.C 17.78,38.1 19.05,39.37 19.05,53.98 SV6.2
N$24
  Top 0.305: S1.1 74.75,61.25 74.75,67.5 S1.2
  Bottom 0.305: TB1.2 70,65.75 71.75,67.5 74.5,67.5 S1.2
N$25
  Top 0.203: D8.C 31.75,57.15 SV8.2
N$26  (via drill 0.35)
  Top 0.203: D9.C 36.83,57.15 v38.1,58.42
  Bottom 0.203: v38.1,58.42 SV9.2
N$27
  Top 0.203: D10.C 44.45,38.1 48.26,41.91 48.26,55.24 SV10.2
N$28
  Top 0.305: S1.4 79.25,67.5 79.25,61.25 S1.3
  Bottom 0.305: TB1.1 70,63 71.25,61.75 73.25,61.75 74,62.5 77.75,62.5 79,61.25 S1.3
N$29
  Bottom 0.305: TB1.3 72.5,63.25 82,63.25 TLED1.A
N$30
  Bottom 0.305: TB1.4 72.5,65.75 82,65.75 TLED1.K
N$31
  Top 0.305: S2.1 74.75,52 74.75,58.25 S2.2
  Bottom 0.305: TB2.2 70,56.75 71.5,58.25 74.5,58.25 S2.2
N$32
  Top 0.305: S2.4 79.25,58.25 79.25,52 S2.3
  Bottom 0.305: TB2.1 70,53.75 71,52.75 73.5,52.75 74.25,53.5 77.5,53.5 79,52 S2.3
N$33
  Bottom 0.305: TB2.3 72.5,54 82,54 TLED2.A
N$34
  Bottom 0.305: TB2.4 72.5,56.5 82,56.5 TLED2.K
N$35  (via drill 0.35)
  Top 0.203: BUT10.1 13.97,6.35 v13.97,12.7 15.24,13.97 D1.A
  Bottom 0.203: IC1.3 45.72,11.43 45.09,12.06 36.2,12.06 35.56,12.7 32.52,12.7 31.6,11.79 21.23,11.79 20.32,12.7 v13.97,12.7
N$36
  Top 0.305: S3.1 74.75,43 74.75,49.25 S3.2
  Bottom 0.305: TB3.2 70,47.5 71.75,49.25 74.5,49.25 S3.2
N$37
  Top 0.305: S3.4 79.25,49.25 79.25,43 S3.3
  Bottom 0.305: TB3.1 70,44.75 73.25,41.5 77.75,41.5 79,42.75 S3.3
N$38
  Bottom 0.305: TB3.3 72.5,44.75 82,44.75 TLED3.A
N$39
  Bottom 0.305: TB3.4 72.5,47.25 82,47.25 TLED3.K
N$40
  Top 0.305: S4.1 74.75,33.75 74.75,40 S4.2
  Bottom 0.305: TB4.2 71.75,40 74.5,40 S4.2
N$41
  Top 0.305: S4.4 79.25,40 79.25,33.75 S4.3
  Bottom 0.305: TB4.1 70,35.5 73.25,32.25 77.75,32.25 79,33.5 S4.3
N$42
  Bottom 0.305: TB4.3 72.5,35.5 82,35.5 TLED4.A
N$43
  Bottom 0.305: TB4.4 72.5,38.25 82,38.25 TLED4.K
N$44
  Top 0.305: S5.1 74.75,24.5 74.75,30.75 S5.2
  Bottom 0.305: TB5.2 70,29 71.75,30.75 74.5,30.75 S5.2
N$45  (via drill 0.35)
  Top 0.203: SV1.6 13.97,48.26 11.43,45.72 W1.8
  Top 0.254: SV1.6 14.61,49.85 v15.24,50.48
  Bottom 0.254: v15.24,50.48 O1.2 | SV1.6 15.88,46.99 22.54,46.99 SV2.4
N$46  (via drill 0.35)
  Top 0.203: SV2.6 22.86,48.26 20.32,45.72 20.32,33.02 W1.5
  Top 0.254: SV2.6 23.81,50.16 v24.13,50.48
  Bottom 0.254: v24.13,50.48 O2.2 | SV2.6 25.08,46.99 31.75,46.99 SV3.4
N$47
  Top 0.305: S5.4 79.25,30.75 79.25,24.5 S5.3
  Bottom 0.305: TB5.1 70,26.25 71.25,25 73.25,25 74,25.75 77.75,25.75 79,24.5 S5.3
N$48
  Bottom 0.305: TB5.3 72.5,26.5 82,26.5 TLED5.A
N$49  (via drill 0.35)
  Top 0.203: W2.8 22.86,40.29 25.08,42.52 25.08,49.87 v25.4,50.19
  Top 0.254: SV4.6 42.23,50.16 v41.91,50.48
  Bottom 0.203: v41.91,50.48 35.88,50.48 35.56,50.17 28.95,50.17 28.93,50.19 v25.4,50.19
  Bottom 0.254: v41.91,50.48 O4.2 | SV4.6 43.5,46.99 50.16,46.99 SV5.4
N$50
  Bottom 0.305: TB5.4 72.5,29 82,29 TLED5.K
N$51  (via drill 0.35)
  Top 0.203: v29.21,50.8 29.21,35.56 27.94,34.29 W2.6 | SV3.6 33.02,49.53 v34.61,51.12
  Bottom 0.203: v34.61,51.12 33.52,51.12 O3.2 32.84,51.44 29.84,51.44 v29.21,50.8
  Bottom 0.254: SV3.6 34.29,46.99 40.96,46.99 SV4.4
N$52
  Top 0.305: S6.1 90,61.25 90,67.5 S6.2
  Bottom 0.305: TB6.2 85.25,65.75 87,67.5 89.75,67.5 S6.2
N$53
  Top 0.305: S6.4 94.5,67.5 94.5,61.25 S6.3
  Bottom 0.305: TB6.1 85.25,63 86.5,61.75 88.5,61.75 89.25,62.5 93,62.5 94.25,61.25 S6.3
N$54
  Top 0.203: SV6.6 14.61,64.14 17.78,67.31 39.37,67.31 40.64,66.04 W3.6
  Bottom 0.203: SV6.6 14.61,64.95 O6.2
  Bottom 0.254: SV6.6 15.88,62.23 22.54,62.23 SV7.4
N$55
  Bottom 0.305: TB6.3 87.75,63.25 97.25,63.25 TLED6.A
N$56  (via drill 0.35)
  Top 0.203: SV7.6 25.74,65.43 v26.04,65.43 | SV8.4 34.29,59.69 34.29,54.61 35.56,53.34 35.56,50.8 34.29,49.53 34.29,39.37 35.56,38.1 W3.8
  Bottom 0.203: v26.04,65.43 24.29,65.43 O7.2
  Bottom 0.254: SV7.6 25.08,62.23 31.75,62.23 SV8.4
N$57  (via drill 0.35)
  Top 0.203: SV8.6 34.92,65.41 v34.92,65.43 | SV9.4 43.5,62.23 43.5,64.22 44.25,64.97 45.17,64.97 46.74,63.4 46.74,41.66 43.18,38.1 W3.5
  Bottom 0.203: v34.92,65.43 33.18,65.43 O8.2
  Bottom 0.254: SV8.6 34.29,62.23 40.96,62.23 SV9.4
N$58  (via drill 0.35)
  Top 0.203: SV9.6 43.81,65.09 v43.81,65.43
  Bottom 0.203: v43.81,65.43 42.07,65.43 O9.2 | SV10.4 52.7,62.23 55.2,62.23 | 55.2,62.23 55.24,62.23 | 55.2,62.23 59.37,58.06 R2.2
  Bottom 0.254: SV9.6 43.5,62.23 50.16,62.23 SV10.4
N$59
  Bottom 0.305: TB6.4 87.75,65.75 97.25,65.75 TLED6.K
N$60
  Top 0.305: S7.1 90,52 90,58.25 S7.2
  Bottom 0.305: TB7.2 85.25,56.75 86.75,58.25 89.75,58.25 S7.2
N$61
  Top 0.305: S7.4 94.5,58.25 94.5,52 S7.3
  Bottom 0.305: TB7.1 85.25,53.75 86.25,52.75 88.75,52.75 89.5,53.5 92.75,53.5 94.25,52 S7.3
N$62
  Bottom 0.305: TB7.3 87.75,54 97.25,54 TLED7.A
N$63
  Bottom 0.305: TB7.4 87.75,56.5 97.25,56.5 TLED7.K
N$64
  Top 0.305: S8.1 90,43 90,49.25 S8.2
  Bottom 0.305: TB8.2 85.25,47.5 87,49.25 89.75,49.25 S8.2
N$65
  Top 0.305: S8.4 94.5,49.25 94.5,43 S8.3
  Bottom 0.305: TB8.1 85.25,44.75 88.5,41.5 93,41.5 94.25,42.75 S8.3
N$66
  Bottom 0.305: TB8.3 87.75,44.75 97.25,44.75 TLED8.A
N$67
  Bottom 0.305: TB8.4 87.75,47.25 97.25,47.25 TLED8.K
N$68
  Top 0.305: S9.1 90,33.75 90,40 S9.2
  Bottom 0.305: TB9.2 85.25,38.25 87,40 89.75,40 S9.2
N$69
  Top 0.305: S9.4 94.5,40 94.5,33.75 S9.3
  Bottom 0.305: TB9.1 85.25,35.5 88.5,32.25 93,32.25 94.25,33.5 S9.3
N$70
  Bottom 0.305: TB9.3 87.75,35.5 97.25,35.5 TLED9.A
N$71
  Bottom 0.305: TB9.4 87.75,38.25 97.25,38.25 TLED9.K
N$72
  Top 0.305: S10.1 90,24.5 90,30.75 S10.2
  Bottom 0.305: TB10.2 85.25,29 87,30.75 89.75,30.75 S10.2
N$73
  Top 0.305: S10.4 94.5,30.75 94.5,24.5 S10.3
  Bottom 0.305: TB10.1 85.25,26.25 86.5,25 88.5,25 89.25,25.75 93,25.75 94.25,24.5 S10.3
N$74
  Bottom 0.305: TB10.3 87.75,26.5 97.25,26.5 TLED10.A
N$75
  Bottom 0.305: TB10.4 87.75,29 97.25,29 TLED10.K
O6
  Top 0.203: SV7.2 27.94,54.29 27.94,39.37 24,35.43 24,28.7 D7.C
RESERVE  (via drill 0.35)
  Top 0.203: v50.8,36.83 52.26,35.37 53,35.37 59.69,28.68 OUTP.8
  Bottom 0.203: v50.8,36.83 41.14,36.83 40.51,36.2 34.03,36.2 33.4,36.83 11.43,36.83 10.16,35.56 10.16,29.21 INP.8
RESET
  Top 0.203: IC1.15 48.26,5.08 54.61,11.43 IC2.8 IC2.9
  Bottom 0.203: IC1.15 47.67,2.54 46.1,4.12 42.41,4.12 42.06,4.47 35.4,4.47 34.44,5.44 29.21,5.44 28.6,6.04 27.32,6.04 26.99,5.71 26.99,4.94 25.91,3.86 13.92,3.86 6.35,11.43 3.81,11.43 2.54,12.7 2.54,19.05 INP.6
RESET_OUT
  Bottom 0.203: IC2.11 55.52,20.68 58.22,20.68 58.58,20.32 OUTP.6
RETURN
  Bottom 0.203: END.1 59.69,12.25 OUTP.2 44.41,15.24 43.65,14.48 35.09,14.48 34.33,15.24 31.71,15.24 30.9,14.43 7.67,14.43 7.34,14.1 4.95,14.1 INP.2

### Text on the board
Top: Top Layer
Bottom: BOTTOM Layer
tPlace: Push Button / Action 4017 | 04.11.19 / V 1.1 | Kai & Hardi | 04.11.19 V 1.1 | Kai & Hardi | Read keyboard matrix
bPlace: Kai & Hardi | Push Button / Action 4017 | +
tNames: Cut here if used to read a keyboard matrix

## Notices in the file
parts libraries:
SparkFun-Retired: Licensing:Creative Commons ShareAlike 4.0 International - https://creativecommons.org/licenses/by-sa/4.0
